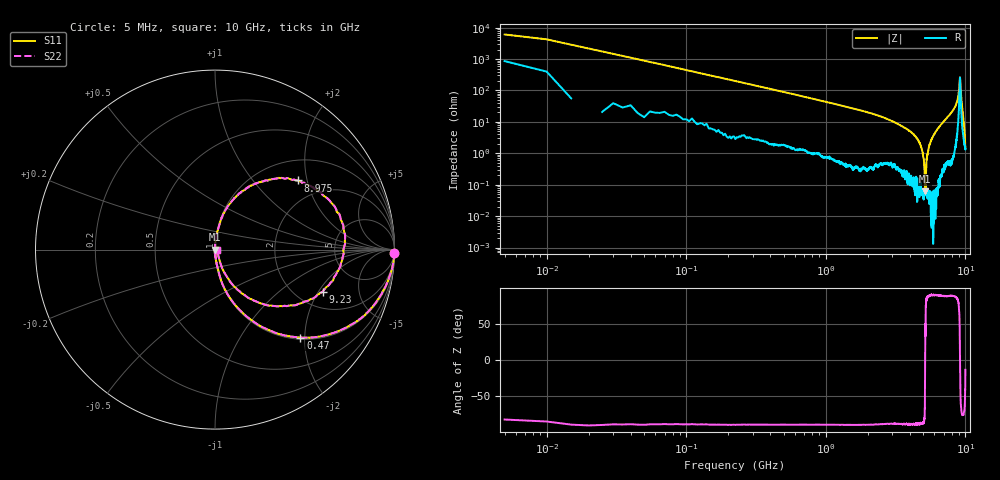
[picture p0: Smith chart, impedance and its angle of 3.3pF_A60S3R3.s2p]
! Amotech Co.,Ltd.
! http://www.amotech.co.kr/
! Part Number: A60S3R3
! These Parameters are Measured in Series Mode Connection
! Operation Temp=25[degC], DC Bias Voltage=0[V]
! Freq. Start=5[MHz] Stop=10[GHz], 2000[Steps]
! Date: Monday, July 13, 2020, 01:27:12
# GHZ S RI R 50.000000
!Freq.(Hz) S11(Real) S11(Imag) S21(Real) S21(Imag) S12(Real) S12(Imag) S22(Real) S22(Imag)
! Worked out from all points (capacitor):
!   2000 points, 5 MHz to 10 GHz, reference 50 ohm
!   read as one part in series: C = 3.58 pF near 55 MHz
!   lowest |Z| = 62.5 mohm at 5.145 GHz (marker M1)
!   series resonance near 5.153 GHz, so ESL is about 270 pH
!   S11 on the Smith chart (normalised r, x): 5 MHz: open; 470 MHz: 1.04, -1.90; 8.975 GHz: 1.46, +1.76; 9.23 GHz: 2.72, -2.18; 10 GHz: 1.03, -0.01
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0.005  0.9974 -0.0162  0.0026 0.0162  0.0026 0.0162  0.9974 -0.0162
0.075  0.9679 -0.1626  0.0321 0.1626  0.0321 0.1626  0.9679 -0.1626
0.14  0.9046 -0.2805  0.0954 0.2805  0.0954 0.2805  0.9046 -0.2805
0.47  0.4761 -0.49  0.5239 0.49  0.5239 0.49  0.4761 -0.49
0.93  0.1857 -0.3801  0.8143 0.3801  0.8143 0.3801  0.1857 -0.3801
1.675  0.061 -0.2319  0.939 0.2319  0.939 0.2319  0.061 -0.2319
3.34  0.00968 -0.0806  0.9903 0.0806  0.9903 0.0806  0.00968 -0.0806
4.545  0.00139 -0.0283  0.9986 0.0283  0.9986 0.0283  0.00139 -0.0283
5.005  0.000566 -0.00727  0.9994 0.00727  0.9994 0.00727  0.000566 -0.00727
5.145  0.000589 -0.000206  0.9994 0.000206  0.9994 0.000206  0.000589 -0.000206
5.185  0.000654 0.000968  0.9993 -0.000968  0.9993 -0.000968  0.000654 0.000968
5.295  0.000552 0.00696  0.9994 -0.00696  0.9994 -0.00696  0.000552 0.00696
5.505  0.000924 0.0174  0.9991 -0.0174  0.9991 -0.0174  0.000924 0.0174
6.67  0.00839 0.0796  0.9916 -0.0796  0.9916 -0.0796  0.00839 0.0796
8.335  0.0782 0.2506  0.9218 -0.2506  0.9218 -0.2506  0.0782 0.2506
8.735  0.1933 0.3549  0.8067 -0.3549  0.8067 -0.3549  0.1933 0.3549
8.975  0.4614 0.3851  0.5386 -0.3851  0.5386 -0.3851  0.4614 0.3851
9.135  0.7251 0.0656  0.2749 -0.0656  0.2749 -0.0656  0.7251 0.0656
9.23  0.5995 -0.2348  0.4005 0.2348  0.4005 0.2348  0.5995 -0.2348
9.495  0.1189 -0.2169  0.8811 0.2169  0.8811 0.2169  0.1189 -0.2169
9.805  0.0249 -0.0599  0.9751 0.0599  0.9751 0.0599  0.0249 -0.0599
10  0.0133 -0.00311  0.9867 0.00311  0.9867 0.00311  0.0133 -0.00311
